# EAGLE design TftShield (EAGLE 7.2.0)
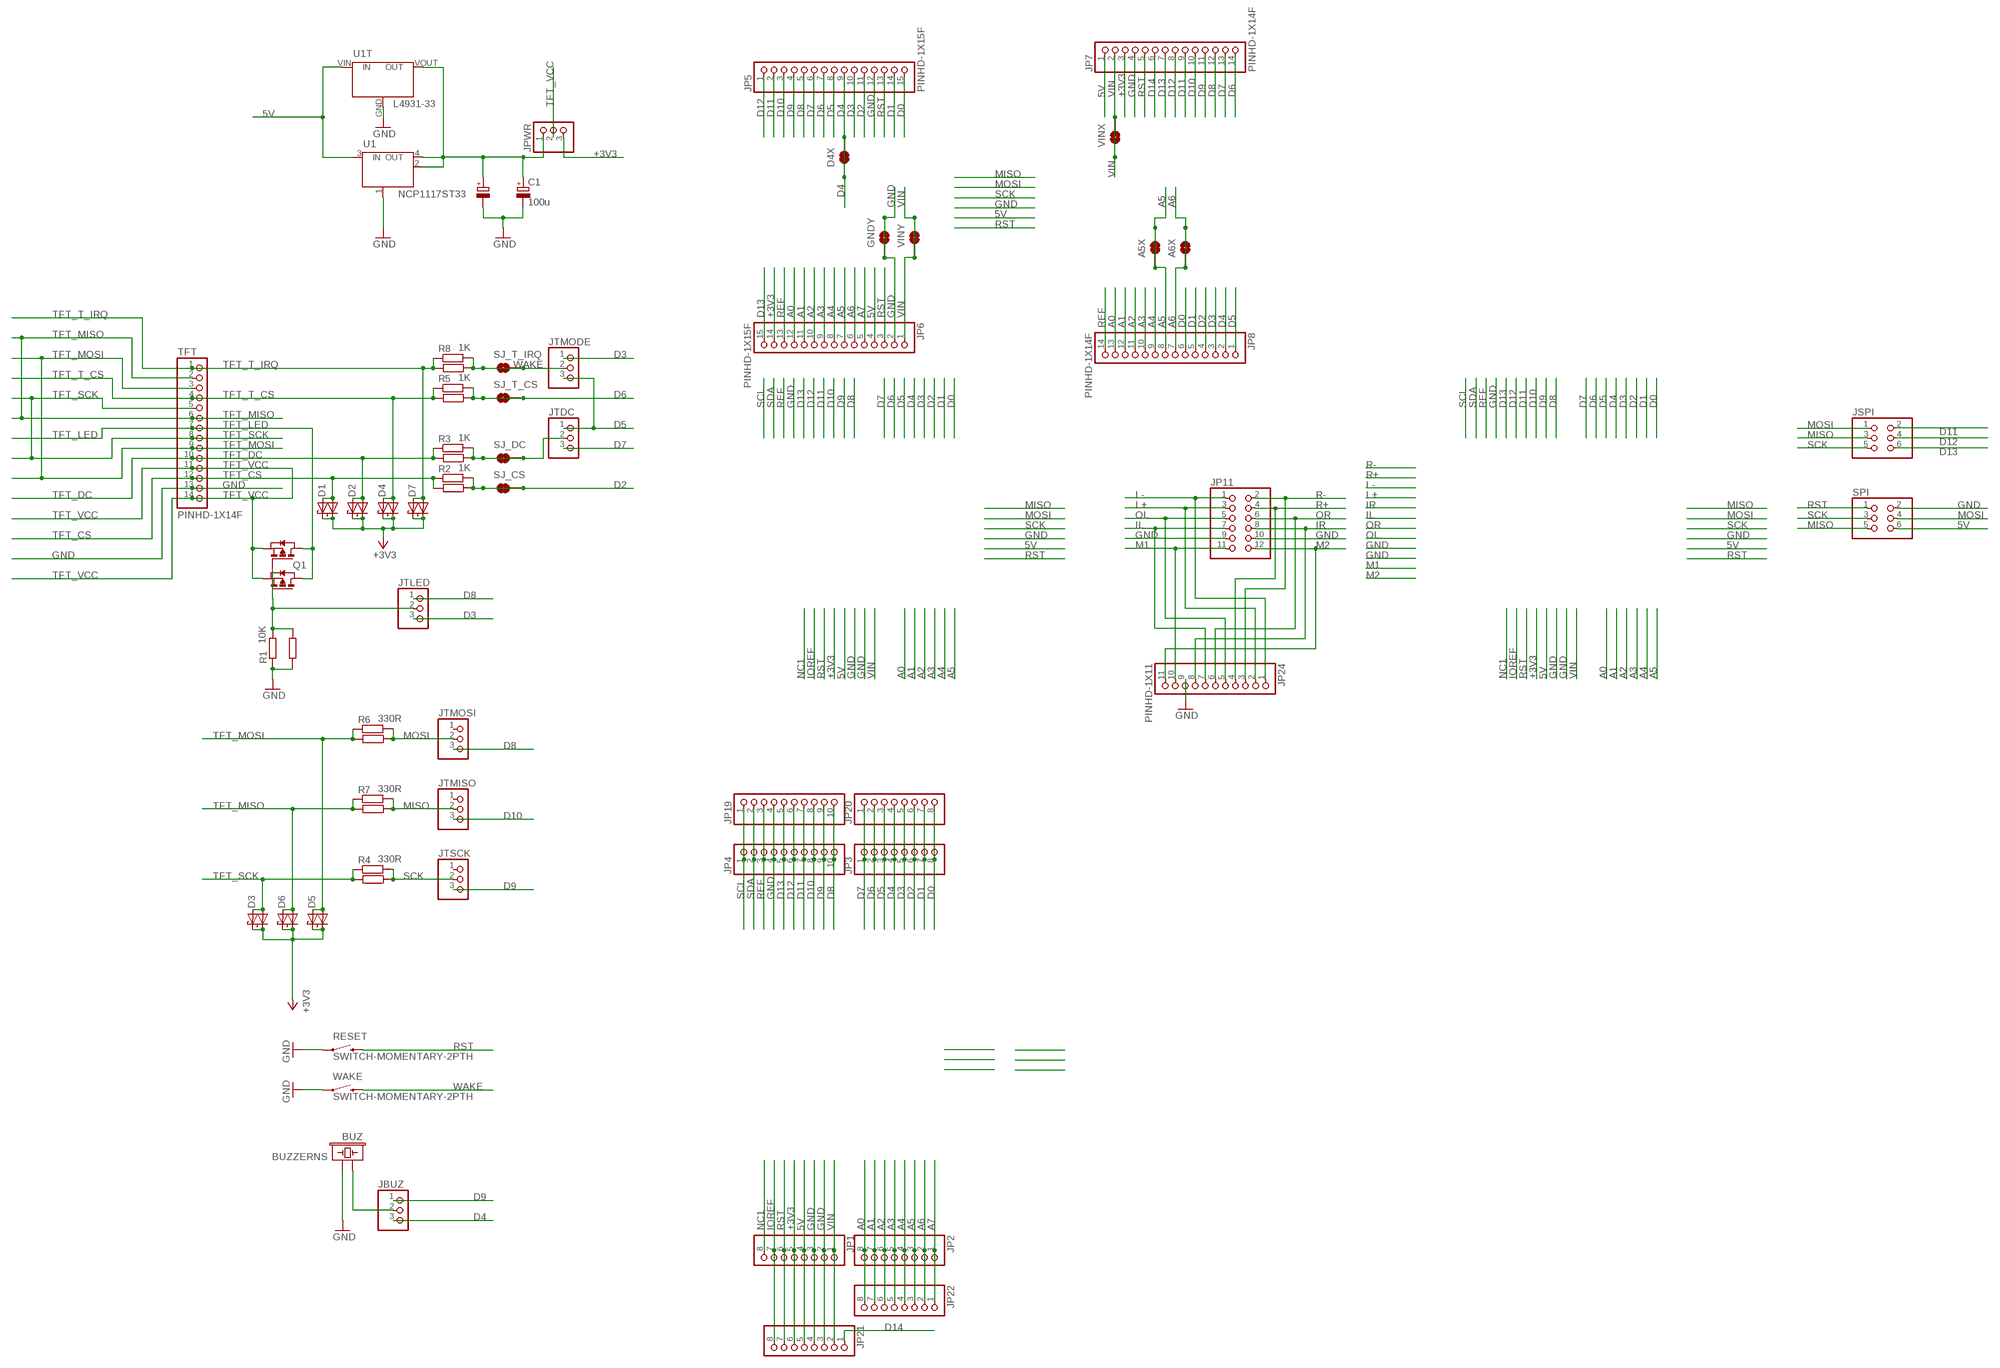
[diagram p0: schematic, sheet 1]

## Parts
A5X  JUMPER-PAD-2-NOYES_SILK  [PAD-JUMPER-2-NO_YES_SILK]
A6X  JUMPER-PAD-2-NOYES_SILK  [PAD-JUMPER-2-NO_YES_SILK]
BUZ  BUZZERNS  [BUZZER-12MM-NS]
C1  100u  CPOLPANASONIC_E  [PANASONIC_E]
C1T  CPOL-EUE3.5-8  [E3,5-8]
D1  RB521S  [SOD523]
D1T  1N4148DO35-7  [DO35-7]
D2  RB521S  [SOD523]
D2T  1N4148DO35-7  [DO35-7]
D3  RB521S  [SOD523]
D3T  1N4148DO35-7  [DO35-7]
D4  RB521S  [SOD523]
D4T  1N4148DO35-7  [DO35-7]
D4X  JUMPER-PAD-2-NOYES_SILK  [PAD-JUMPER-2-NO_YES_SILK]
D5  RB521S  [SOD523]
D5T  1N4148DO35-7  [DO35-7]
D6  RB521S  [SOD523]
D6T  1N4148DO35-7  [DO35-7]
D7  RB521S  [SOD523]
D7T  1N4148DO35-7  [DO35-7]
GNDY  JUMPER-PAD-2-NOYES_SILK  [PAD-JUMPER-2-NO_YES_SILK]
JBUZ  PINHD-1X3  [1X03M]
JP1  PINHD-1X8  [1X08M]
JP2  PINHD-1X8  [1X08M]
JP3  PINHD-1X8  [1X08M]
JP4  PINHD-1X10  [1X10M]
JP5  PINHD-1X15F  [1X15F]
JP6  PINHD-1X15F  [1X15F]
JP7  PINHD-1X14F  [1X14F]
JP8  PINHD-1X14F  [1X14F]
JP11  PINHD-2X6F  [2X06F]
JP19  PINHD-1X10  [1X10M]
JP20  PINHD-1X8  [1X08M]
JP21  PINHD-1X8  [1X08M]
JP22  PINHD-1X8  [1X08M]
JP24  PINHD-1X11  [1X11M]
JPWR  PINHD-1X3  [1X03M]
JSPI  PINHD-2X3  [2X03M]
JTDC  PINHD-1X3  [1X03M]
JTLED  PINHD-1X3  [1X03M]
JTMISO  PINHD-1X3  [1X03M]
JTMODE  PINHD-1X3  [1X03M]
JTMOSI  PINHD-1X3  [1X03M]
JTSCK  PINHD-1X3  [1X03M]
Q1  PMOSSOT23  [SOT23]
Q1T  BS170  [TO92-MOSFET]
R1  10K  R0603-ROUND  [R0603-ROUND]
R1T  R0204-5  [0204-5]
R2  1K  R0603-ROUND  [R0603-ROUND]
R2T  R0204-5  [0204-5]
R3  1K  R0603-ROUND  [R0603-ROUND]
R3T  R0204-5  [0204-5]
R4  330R  R0603-ROUND  [R0603-ROUND]
R4T  R0204-5  [0204-5]
R5  1K  R0603-ROUND  [R0603-ROUND]
R5T  R0204-5  [0204-5]
R6  330R  R0603-ROUND  [R0603-ROUND]
R6T  R0204-5  [0204-5]
R7  330R  R0603-ROUND  [R0603-ROUND]
R7T  R0204-5  [0204-5]
R8  1K  R0603-ROUND  [R0603-ROUND]
R8T  R0204-5  [0204-5]
RESET  SWITCH-MOMENTARY-2PTH  [TACTILE-PTH]
SJ_CS  JUMPER-PAD-2-NOYES_SILK  [PAD-JUMPER-2-NO_YES_SILK]
SJ_DC  JUMPER-PAD-2-NOYES_SILK  [PAD-JUMPER-2-NO_YES_SILK]
SJ_T_CS  JUMPER-PAD-2-NOYES_SILK  [PAD-JUMPER-2-NO_YES_SILK]
SJ_T_IRQ  JUMPER-PAD-2-NOYES_SILK  [PAD-JUMPER-2-NO_YES_SILK]
SPI  PINHD-2X3F  [2X03F]
TFT  PINHD-1X14F  [1X14F]
U1  NCP1117ST33  [SOT223]
U1T  L4931-33  [TO92]
VINX  JUMPER-PAD-2-NOYES_SILK  [PAD-JUMPER-2-NO_YES_SILK]
VINY  JUMPER-PAD-2-NOYES_SILK  [PAD-JUMPER-2-NO_YES_SILK]
WAKE  SWITCH-MOMENTARY-2PTH  [TACTILE-PTH]

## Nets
5V: JP1.4 JP6.4 JP7.1 JP21.5 SPI.6 U1.3(IN) U1T.VIN(IN)
+3V3: D1.C D1T.C D2.C D2T.C D3.C D3T.C D4.C D4T.C D5.C D5T.C D6.C D6T.C D7.C D7T.C JP1.5 JP6.14 JP7.3 JP21.6 JPWR.3
A0: JP2.8 JP6.12 JP8.13 JP22.8
A1: JP2.7 JP6.11 JP8.12 JP22.7
A2: JP2.6 JP6.10 JP8.11 JP22.6
A3: JP2.5 JP6.9 JP8.10 JP22.5
A4: JP2.4 JP6.8 JP8.9 JP22.4
A5: A5X.1 A5X.2 JP2.3 JP6.7 JP8.8 JP22.3
A6: A6X.1 A6X.2 JP2.2 JP6.6 JP8.7 JP22.2
A7: JP2.1 JP6.5 JP22.1
D0: JP3.8 JP5.15 JP8.6 JP20.8
D1: JP3.7 JP5.14 JP8.5 JP20.7
D2: JP3.6 JP5.11 JP8.4 JP20.6 R2.2 R2T.1 SJ_CS.1 SJ_CS.2
D3: JP3.5 JP5.10 JP8.3 JP20.5 JTLED.3 JTMODE.1
D4: D4X.1 D4X.2 JBUZ.3 JP3.4 JP5.9 JP8.2 JP20.4
D5: JP3.3 JP5.8 JP8.1 JP20.3 JTDC.1 JTMODE.3
D6: JP3.2 JP5.7 JP7.14 JP20.2 R5.2 R5T.1 SJ_T_CS.1 SJ_T_CS.2
D7: JP3.1 JP5.6 JP7.13 JP20.1 JTDC.3
D8: JP4.10 JP5.5 JP7.12 JP19.10 JTLED.1 JTMOSI.3
D9: JBUZ.1 JP4.9 JP5.4 JP7.11 JP19.9 JTSCK.3
D10: JP4.8 JP5.3 JP7.10 JP19.8 JTMISO.3
D11: JP4.7 JP5.2 JP7.9 JP19.7 JSPI.2
D12: JP4.6 JP5.1 JP7.8 JP19.6 JSPI.4
D13: JP4.5 JP6.15 JP7.7 JP19.5 JSPI.6
D14: JP7.6 JP21.1
GND: BUZ.- C1.- C1T.- GNDY.1 GNDY.2 JP1.2 JP1.3 JP4.4 JP5.12 JP6.2 JP7.4 JP11.9 JP11.10 JP19.4 JP21.3 JP21.4 JP24.9 R1.1 R1T.1 RESET.1 RESET.2 SPI.2 TFT.13 U1.1(GND/ADJ) U1T.GND(GND/ADJ) WAKE.1 WAKE.2
IL: JP11.7 JP24.7
IOREF: JP1.7 JP21.8
IR: JP11.8 JP24.8
L+: JP11.3 JP24.2
L-: JP11.1 JP24.1
M1: JP11.11 JP24.10
M2: JP11.12 JP24.11
MISO: JSPI.3 JTMISO.2 R7.2 R7T.1 SPI.5
MOSI: JSPI.1 JTMOSI.2 R6.2 R6T.1 SPI.4
N$2: BUZ.+ JBUZ.2
N$4: JTLED.2 Q1.1(G) Q1T.G R1.2 R1T.2
N$5: JTDC.2 R3.2 R3T.1 SJ_DC.1 SJ_DC.2
N$10: C1.+ C1T.+ JPWR.1 U1.2(OUT) U1.4(OUT) U1T.VOUT(OUT)
NC1: JP1.8
OL: JP11.5 JP24.5
OR: JP11.6 JP24.6
R+: JP11.4 JP24.4
R-: JP11.2 JP24.3
REF: JP4.3 JP6.13 JP8.14 JP19.3
RST: JP1.6 JP5.13 JP6.3 JP7.5 JP21.7 RESET.3 RESET.4 SPI.1
SCK: JSPI.5 JTSCK.2 R4.2 R4T.1 SPI.3
SCL: JP4.1 JP19.1
SDA: JP4.2 JP19.2
TFT_CS: D1.A D1T.A R2.1 R2T.2 TFT.12
TFT_DC: D2.A D2T.A R3.1 R3T.2 TFT.10
TFT_LED: Q1.3(D) Q1T.D TFT.7
TFT_MISO: D6.A D6T.A R7.1 R7T.2 TFT.2 TFT.6
TFT_MOSI: D5.A D5T.A R6.1 R6T.2 TFT.3 TFT.9
TFT_SCK: D3.A D3T.A R4.1 R4T.2 TFT.5 TFT.8
TFT_T_CS: D4.A D4T.A R5.1 R5T.2 TFT.4
TFT_T_IRQ: D7.A D7T.A R8.1 R8T.2 TFT.1
TFT_VCC: JPWR.2 Q1.2(S) Q1T.S TFT.11 TFT.14
VIN: JP1.1 JP6.1 JP7.2 JP21.2 VINX.1 VINX.2 VINY.1 VINY.2
WAKE: JTMODE.2 R8.2 R8T.1 SJ_T_IRQ.1 SJ_T_IRQ.2 WAKE.3 WAKE.4
Unconnected: JTMISO.1 JTMOSI.1 JTSCK.1

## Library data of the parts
A5X A6X D4X GNDY SJ_CS SJ_DC SJ_T_CS SJ_T_IRQ VINX VINY = Max-Connectors:JUMPER-PAD-2-NO
BUZ = Max-Buzzers:BUZZER: Buzzer 12mm
C1 = Max-RCL:CPOL
C1T = rcl:CPOL-EU: POLARIZED CAPACITOR, European symbol
D1-D7 = Max-Diodes:RB521S
D1T D2T D3T D4T D5T D6T D7T = Max-Diodes:1N4148: DIODE
JBUZ JPWR JTDC JTLED JTMISO JTMODE JTMOSI JTSCK = Max-PinHead:PINHD-1X3: PIN HEADER
JP1-JP3 JP20-JP22 = Max-PinHead:PINHD-1X8: PIN HEADER
JP4 JP19 = Max-PinHead:PINHD-1X10: PIN HEADER
JP5 JP6 = Max-PinHead:PINHD-1X15
JP7 JP8 TFT = Max-PinHead:PINHD-1X14
JP11 = Max-PinHead:PINHD-2X6
JP24 = Max-PinHead:PINHD-1X11
JSPI SPI = Max-PinHead:PINHD-2X3: PIN HEADER
Q1 = Max-Mosfets:PMOSSOT23: MOS FET
Q1T = Max-Mosfets:BS170
R1 R1T R2 R2T R3 R3T R4 R4T R5 R5T R6 R6T R7 R7T R8 R8T = Max-RCL:R
RESET WAKE = Max-Switches:SWITCH-MOMENTARY-2: Various NO switches- pushbuttons, reed, etc; PROD_ID: SWCH-08441
U1 = Max-LinearRegulators:NCP1117: Adjustable Output Low Dropout Voltage Regulator 800 mA Source: http://www.onsemi.com/pub/Collateral/MC33269-D.PDF
U1T = Max-LinearRegulators:L4931-33

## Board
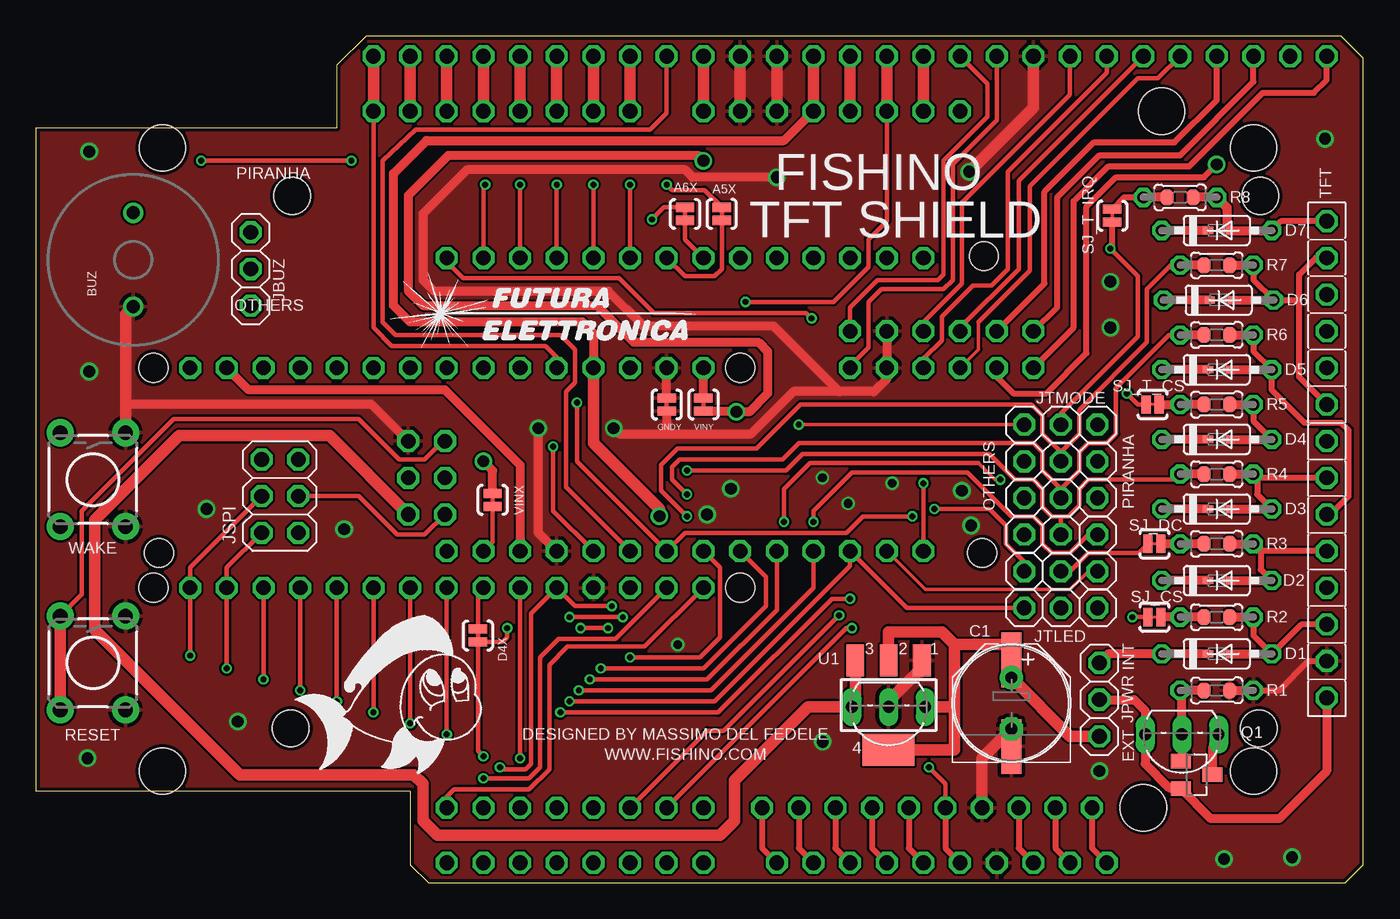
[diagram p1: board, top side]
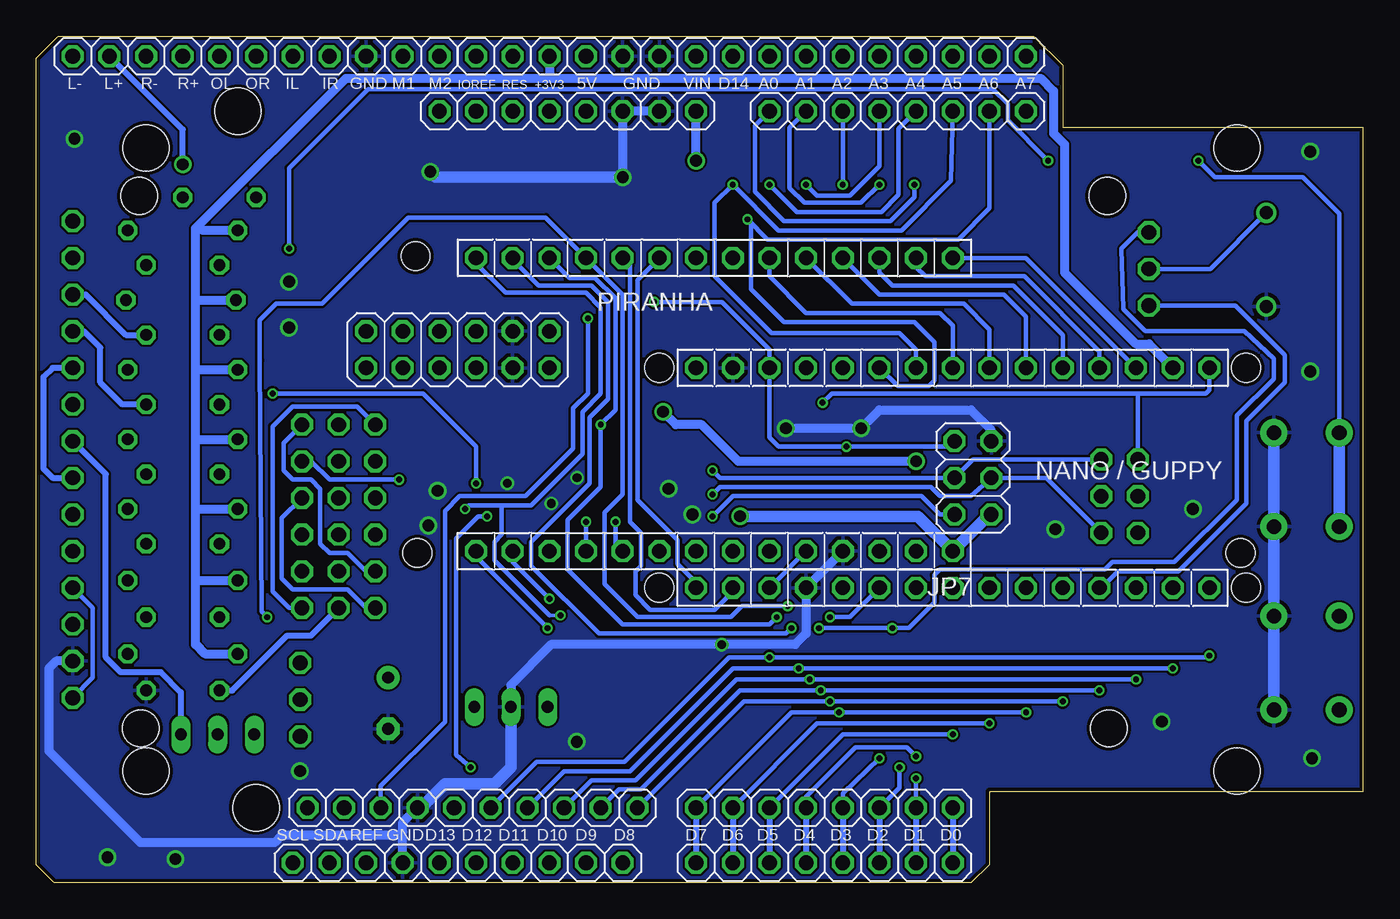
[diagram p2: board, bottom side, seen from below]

Size 91.95 x 58.67 mm. Coordinates in mm from the lower left corner, seen from the top.
Outline: 25.91,6.35 25.91,1.27 27.18,0 90.68,0 91.95,1.27 91.95,57.15 90.42,58.67 22.86,58.67 20.83,56.64 20.83,52.32 0,52.32 0,6.35 25.91,6.35
Copper layers (1*16): Top 0.035mm / dielectric 1.5mm / Bottom 0.035mm
Design rules "Elecrow_2-layer_eagle_rule": minimum track width 6mil, minimum drill 12mil, track to track 6mil, track to pad 6mil, pad to pad 6mil, via to via 6mil, smd to smd 0mil, copper to edge 10mil, drill to drill 10mil, minimum pad ring 10mil, minimum via ring 6mil, stop-mask expansion 2mil, vias tented up to drill 100mil, thermal gap 10mil
Holes 3.2 mm at 84.33,7.75 8.76,7.75 8.76,50.93 84.33,50.93 76.71,5.21 77.98,53.47
Holes 2 mm at 8.13,20.45 8.51,22.86 8.13,35.69 48.77,20.45 48.77,35.69 65.53,22.86 65.66,43.43
Holes 2.54 mm at 17.73,47.6 17.63,10.72 84.71,10.72 84.81,47.6

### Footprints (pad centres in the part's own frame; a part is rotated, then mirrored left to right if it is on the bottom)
PAD-JUMPER-2-NO_YES_SILK = smd 0.635 x 1.27: 1 -0.45,0; 2 0.45,0
BUZZER-12MM-NS = drill 0.9: + 3.25,0; - -3.25,0
PANASONIC_E = smd 3.8 x 1.4: + 3,0; - -3,0
E3,5-8 = drill 0.813 pad 1.6: + -1.778,0 | drill 0.813 pad 1.6 octagon: - 1.778,0
SOD523 = smd 0.7 x 0.5: A 0.7,0; C -0.6,0
DO35-7 = drill 0.813 octagon: A 3.81,0; C -3.81,0
1X03M = drill 1.016 octagon: 1 -2.54,0; 2 0,0; 3 2.54,0
1X08M = drill 1.016 octagon: 1 -8.89,0; 2 -6.35,0; 3 -3.81,0; 4 -1.27,0; 5 1.27,0; 6 3.81,0; 7 6.35,0; 8 8.89,0
1X10M = drill 1.016 octagon: 1 -11.43,0; 2 -8.89,0; 3 -6.35,0; 4 -3.81,0; 5 -1.27,0; 6 1.27,0; 7 3.81,0; 8 6.35,0; 9 8.89,0; 10 11.43,0
1X15F = drill 1.016 octagon: 1 -17.78,0; 2 -15.24,0; 3 -12.7,0; 4 -10.16,0; 5 -7.62,0; 6 -5.08,0; 7 -2.54,0; 8 0,0; 9 2.54,0; 10 5.08,0; 11 7.62,0; 12 10.16,0; 13 12.7,0; 14 15.24,0; 15 17.78,0
1X14F = drill 1.016 octagon: 1 -16.51,0; 2 -13.97,0; 3 -11.43,0; 4 -8.89,0; 5 -6.35,0; 6 -3.81,0; 7 -1.27,0; 8 1.27,0; 9 3.81,0; 10 6.35,0; 11 8.89,0; 12 11.43,0; 13 13.97,0; 14 16.51,0
2X06F = drill 1.016 octagon: 1 -6.35,-1.27; 2 -6.35,1.27; 3 -3.81,-1.27; 4 -3.81,1.27; 5 -1.27,-1.27; 6 -1.27,1.27; 7 1.27,-1.27; 8 1.27,1.27; 9 3.81,-1.27; 10 3.81,1.27; 11 6.35,-1.27; 12 6.35,1.27
1X11M = drill 1.016 octagon: 1 -12.7,0; 2 -10.16,0; 3 -7.62,0; 4 -5.08,0; 5 -2.54,0; 6 0,0; 7 2.54,0; 8 5.08,0; 9 7.62,0; 10 10.16,0; 11 12.7,0
2X03M = drill 1.016 octagon: 1 -2.54,-1.27; 2 -2.54,1.27; 3 0,-1.27; 4 0,1.27; 5 2.54,-1.27; 6 2.54,1.27
SOT23 = smd 1 x 1.4: 1 -0.95,-1.1; 2 0.95,-1.1; 3 0,1.1
TO92-MOSFET = drill 0.813 long: D -2.54,0; G 0,0; S 2.54,0
R0603-ROUND = smd 0.898 x 1.1: 1 -0.889,0; 2 0.889,0
0204-5 = drill 0.813 octagon: 1 -2.54,0; 2 2.54,0
TACTILE-PTH = drill 1.016 pad 1.88: 1 -3.251,2.261; 2 3.251,2.261; 3 -3.251,-2.261; 4 3.251,-2.261
2X03F = drill 1.016 octagon: 1 -2.54,-1.27; 2 -2.54,1.27; 3 0,-1.27; 4 0,1.27; 5 2.54,-1.27; 6 2.54,1.27
SOT223 = smd 1.219 x 2.235: 1 -2.311,-3.099; 2 0,-3.099; 3 2.311,-3.099 | smd 3.6 x 2.2: 4 0,3.099
TO92 = drill 0.813 long: GND 0,0; VIN 2.54,0; VOUT -2.54,0

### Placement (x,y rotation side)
A5X  47.5,46.35 90 top
A6X  44.96,46.35 90 top
BUZ  6.73,43.18 90 top
C1  67.56,12.45 90 top
C1T  67.56,12.45 270 top
D1  81.79,15.88 0 top
D1T  81.79,15.88 0 top
D2  81.79,20.95 0 top
D2T  81.79,20.95 0 top
D3  81.79,25.91 0 top
D3T  81.79,25.91 0 top
D4  81.79,30.73 0 top
D4T  81.79,30.73 0 top
D4X  30.61,17.14 90 top
D5  81.79,35.56 0 top
D5T  81.79,35.56 0 top
D6  81.92,40.39 0 top
D6T  81.92,40.39 0 top
D7  81.79,45.21 0 top
D7T  81.79,45.21 0 top
GNDY  43.69,33.15 270 top
JBUZ  14.86,42.55 90 top
JP1  55.12,53.47 180 bottom
JP2  32.26,53.47 180 bottom
JP3  37.34,5.21 0 bottom
JP4  61.72,5.21 0 bottom
JP5  28.45,20.45 180 bottom
JP6  28.45,35.69 0 bottom
JP7  44.96,22.99 180 bottom
JP8  44.96,43.31 0 bottom
JP11  62.74,36.96 0 bottom
JP19  62.74,1.4 0 bottom
JP20  37.34,1.4 0 bottom
JP21  52.58,57.28 180 bottom
JP22  32.26,57.28 180 bottom
JP24  76.71,57.28 0 bottom
JPWR  73.66,12.7 90 top
JSPI  16.89,26.8 90 top
JTDC  70.99,21.59 0 top
JTLED  70.99,19.05 0 top
JTMISO  70.99,29.21 0 top
JTMODE  70.99,31.75 0 top
JTMOSI  70.99,26.67 0 top
JTSCK  70.99,24.13 0 top
Q1  80.39,7.49 270 top
Q1T  79.38,10.29 180 top
R1  81.79,13.34 180 top
R1T  81.79,13.34 180 top
R2  81.79,18.41 180 top
R2T  81.79,18.41 0 top
R3  81.79,23.5 180 top
R3T  81.79,23.5 0 top
R4  81.79,28.32 180 top
R4T  81.79,28.32 0 top
R5  81.79,33.15 180 top
R5T  81.79,33.15 0 top
R6  81.79,37.97 180 top
R6T  81.79,37.97 0 top
R7  81.79,42.8 180 top
R7T  81.79,42.8 0 top
R8  79.25,47.5 180 top
R8T  79.25,47.5 0 top
RESET  3.94,15.24 270 top
SJ_CS  77.47,18.41 180 top
SJ_DC  77.47,23.5 180 top
SJ_T_CS  77.34,33.15 180 top
SJ_T_IRQ  74.55,46.23 270 top
SPI  27.05,28.07 270 bottom
TFT  89.41,29.34 270 top
U1  59.05,12.32 180 top
U1T  59.05,12.19 180 top
U$3  [FISHINO]  19.68,7.87 0 top
U$5  [FUTURA]  24.38,37.08 0 top
VINX  31.62,26.54 270 top
VINY  46.23,33.15 270 top
WAKE  3.94,27.94 270 top

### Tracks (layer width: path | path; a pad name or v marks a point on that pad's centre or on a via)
5V  (via drill 0.81)
  Top 0.61: JP6.4 38.61,38.1 37.85,38.86 25.91,38.86 24.77,40.01 24.77,49.15 27.05,51.44 51.82,51.44 JP1.4
  Top 0.813: U1.3 56.74,12.42 U1T.VIN 53.47,12.19 48.39,7.11 48.39,4.32 47.37,3.3 27.81,3.3 26.8,4.32 26.8,6.86 26.16,7.49 14.1,7.49 4.06,17.53 4.06,25.15 9.91,30.99 20.32,30.99 SPI.6 | JP1.4 JP21.5 | v43.18,25.4 43.18,25.91 38.61,30.48 JP6.4
  Bottom 0.813: v43.18,25.4 30.86,25.4 JP7.1 25.91,25.53 SPI.6
+3V3
  Top 0.61: JP7.3 33.53,28.96 28.32,34.16 14.73,34.16 JP6.14 | D7.C D7T.C | D6.C D6T.C | D5.C D5T.C | D4.C D4T.C | D3.C D3T.C | D1.C D1T.C 74.3,15.88 JPWR.3 | D2.C D2T.C
  Top 0.813: JP1.5 JP21.6
  Bottom 0.61: 56.39,55.75 22.35,55.75 21.46,54.86 21.46,51.94 20.7,51.18 20.7,42.29 15.75,37.34 14.86,37.34 JP6.14 | D1T.C 80.26,15.88 80.9,16.51 80.9,20.95 | 80.9,20.95 D2T.C | 80.9,20.95 80.9,25.91 | 80.9,25.91 D3T.C | 80.9,25.91 80.9,30.73 | 80.9,30.73 D4T.C | 80.9,30.73 80.9,35.56 | 80.9,35.56 D5T.C | 80.9,35.56 80.9,40.39 | 80.9,40.39 D6T.C | 80.9,40.39 80.9,45.34 80.71,45.53 | JP21.6 56.39,55.75 | D7T.C 80.39,45.21 80.71,45.53 | 80.71,45.53 70.48,55.75 56.39,55.75
A0  (via drill 0.41)
  Top 0.305: JP8.13 30.99,48.26 v31.11,48.39
  Top 0.813: JP2.8 JP22.8
  Bottom 0.305: JP2.8 42.16,52.45 42.16,47.88 40.13,45.85 32.77,45.85 31.11,47.5 v31.11,48.39 | JP8.13 30.99,42.67 30.35,42.04 23.5,42.04 18.29,36.83 JP6.12
A1  (via drill 0.41)
  Top 0.305: JP8.12 v33.53,48.39
  Top 0.813: JP2.7 JP22.7
  Bottom 0.305: JP2.7 39.75,52.32 39.75,48.13 38.73,47.12 34.8,47.12 v33.53,48.39 | JP8.12 33.53,42.29 32.64,41.4 24.26,41.4 20.83,37.97 JP6.11
A2  (via drill 0.41)
  Top 0.305: v36.07,48.39 JP8.11
  Top 0.813: JP2.6 JP22.6
  Bottom 0.305: JP2.6 v36.07,48.39 | JP8.11 33.53,40.77 24.89,40.77 23.37,39.24 JP6.10
A3  (via drill 0.41)
  Top 0.305: JP8.10 v38.61,48.39
  Top 0.813: JP2.5 JP22.5
  Bottom 0.305: JP2.5 33.53,49.66 35.56,47.62 37.85,47.62 v38.61,48.39 | JP6.9 25.91,38.35 27.69,40.13 35.43,40.13 JP8.10
A4  (via drill 0.41)
  Top 0.305: JP8.9 v41.15,48.39
  Top 0.813: JP2.4 JP22.4
  Bottom 0.305: JP2.4 32.19,52.26 32.19,47.69 33.4,46.48 39.24,46.48 v41.15,48.39 | JP6.8 28.45,38.61 29.34,39.5 38.61,39.5 41.15,42.04 JP8.9
A5  (via drill 0.41)
  Top 0.305: v43.69,48.39 44.07,48.01 46.3,48.01 A5X.2 A5X.1 47.5,42.55 46.99,42.04 44.96,42.04 JP8.8
  Top 0.813: JP2.3 JP22.3
  Bottom 0.305: JP2.3 28.57,48.64 32,45.21 40.51,45.21 v43.69,48.39 44.96,47.12 44.96,42.04 41.02,38.1 32.13,38.1 30.99,36.96 JP6.7
A6  (via drill 0.41)
  Top 0.305: v42.67,45.97 43.5,46.8 A6X.2 A6X.1 44.96,44.58 JP8.7
  Top 0.813: JP2.2 JP22.2
  Bottom 0.305: JP2.2 25.91,46.74 28.07,44.58 41.27,44.58 v42.67,45.97 42.42,45.72 42.42,41.15 40.13,38.86 31.11,38.86 29.72,37.47 29.72,34.8 30.1,34.42 32.26,34.42 JP6.6
A7
  Top 0.305: JP6.5 36.07,36.45 35.31,37.21 24.64,37.21 23.37,38.48 JP2.1
  Top 0.813: JP2.1 JP22.1
D0
  Top 0.305: JP5.15 42.16,16.38 36.83,16.38 35.56,15.11 35.56,7.87 34.16,6.48 28.96,6.48 28.45,5.97 JP3.8
  Bottom 0.305: JP5.15 46.23,20.83 47.5,22.1 47.5,23.75 50.29,26.54 50.29,41.78 JP8.6
  Bottom 0.406: JP3.8 JP20.8
D1  (via drill 0.41)
  Top 0.305: v30.99,7.24 34.16,7.24 34.92,8 34.92,15.62 36.2,16.89 40.13,16.89 JP5.14
  Bottom 0.305: JP3.7 v30.99,7.24 | JP5.14 43.69,20.19 44.96,18.92 49.4,18.92 50.42,19.94 50.42,21.59 50.04,21.97 50.04,24.26 50.8,25.02 50.8,42.8 JP8.5
  Bottom 0.406: JP3.7 JP20.7
D2  (via drill 0.41)
  Top 0.203: SJ_CS.2 SJ_CS.1
  Top 0.254: v32.13,8 32.26,7.87
  Top 0.305: 32.26,7.87 33.91,7.87 34.29,8.26 34.29,18.67 JP5.11 37.34,19.18 v39.88,19.18 | SJ_CS.2 v75.95,18.41
  Top 0.61: SJ_CS.1 R2T.1 R2.2
  Bottom 0.305: JP3.6 32.13,6.6 v32.13,8 | v39.88,19.18 43.05,19.18 43.81,18.41 50.29,18.41 52.58,20.7 52.58,25.65 51.31,26.92 51.31,40.77 JP8.4 56.64,46.1 66.17,46.1 72.14,40.13 75.31,40.13 76.45,38.99 76.45,36.2 76.33,18.8 v75.95,18.41
  Bottom 0.406: JP3.6 JP20.6
D3  (via drill 0.41)
  Top 0.254: JTMODE.1 v52.83,31.75
  Top 0.305: v33.53,8.64 JP5.10 | v40.64,18.41 v36.96,18.41
  Bottom 0.305: v33.53,8.64 36.07,6.22 JP3.5 | v40.64,18.41 41.15,17.91 51.31,17.91 55.12,21.72 55.12,25.15 52.83,27.43 v52.83,31.75 51.82,32.77 51.82,40.51 53.21,41.91 54.99,41.91 JP8.3 | v36.96,18.41 35.56,18.41 JP5.10 | JTLED.3 74.42,19.05 75.56,20.19 75.56,31.62 74.17,33.02 69.72,33.02 JTMODE.1
  Bottom 0.406: JP3.5 JP20.5
D4  (via drill 0.41)
  Top 0.305: v39.62,17.65 v37.72,17.65 | D4X.1 30.61,9.14 v30.99,8.76 | D4X.1 32.32,16.7 32.64,17.02 v32.64,17.65 | D4X.1 D4X.2 30.61,20.07 JP5.9
  Bottom 0.305: JP3.4 38.61,5.97 35.18,9.4 31.62,9.4 v30.99,8.76 | JP8.2 58.93,43.18 57.15,41.4 53.47,41.4 52.32,40.26 52.32,33.53 53.59,32.26 53.59,27.69 57.66,23.62 57.66,21.97 52.96,17.27 40.01,17.27 v39.62,17.65 | JBUZ.3 15.62,45.09 16.76,43.94 16.64,39.75 15.11,38.23 8.26,38.23 6.22,36.32 6.22,34.92 8.76,32.38 8.76,26.54 13.08,22.23 17.4,22.23 17.91,21.72 29.34,21.72 29.72,21.34 29.72,19.43 31.5,17.65 v32.64,17.65 v37.72,17.65
  Bottom 0.406: JP3.4 JP20.4
D5  (via drill 0.41)
  Top 0.305: JP5.8 v28.45,10.29 | v55.63,18.54 47.62,10.54 46.48,10.54 JP3.3 | JTDC.1 68.45,22.23 67.18,23.5 67.18,24.77 66.04,25.91 v62.23,25.91
  Bottom 0.254: 56.39,18.54 v55.63,18.54
  Bottom 0.305: v28.45,10.29 36.07,10.29 JP3.3 | JP8.1 61.47,42.93 59.44,40.89 53.85,40.89 52.83,39.88 52.83,33.91 54.1,32.64 54.1,29.72 57.66,26.16 59.69,26.16 | 56.39,18.54 60.2,22.35 60.2,23.62 59.69,24.13 59.69,26.16 | JTDC.1 69.09,21.59 70.36,22.86 71.63,22.86 72.26,23.5 72.26,27.3 72.9,27.94 74.17,27.94 74.8,28.57 74.8,30.48 JTMODE.3 | v62.23,25.91 61.98,26.16 59.69,26.16
  Bottom 0.406: JP3.3 JP20.3
D6  (via drill 0.41)
  Top 0.203: SJ_T_CS.1 SJ_T_CS.2
  Top 0.305: JP5.7 v25.91,11.05 | SJ_T_CS.2 76.33,33.15 v75.56,33.91 | JP3.2 56.13,17.65 v56.52,17.65 | v61.47,27.69 JP7.14
  Top 0.61: R5.2 R5T.1 SJ_T_CS.1
  Bottom 0.305: v25.91,11.05 37.85,11.05 JP3.2 | v75.56,33.91 65.15,33.91 61.47,30.23 v61.47,27.69 | v56.52,17.65 61.47,22.61 JP7.14
  Bottom 0.406: JP3.2 JP20.2
D7  (via drill 0.41)
  Top 0.254: JTDC.3 72.9,21.59 71.63,20.32 61.59,20.32 JP7.13
  Top 0.305: JP5.6 v23.37,11.81 | v56.39,19.68 55.12,19.68 47.24,11.81 v36.32,11.81
  Bottom 0.305: v23.37,11.81 v36.32,11.81 39.62,11.81 JP3.1 | JP7.13 58.93,22.23 v56.39,19.68
  Bottom 0.406: JP3.1 JP20.1
D8  (via drill 0.41)
  Top 0.305: JP5.5 v20.83,12.57 | JTLED.1 60.33,19.05 JP7.12 56.39,21.97 46.99,12.57 v36.96,12.57
  Top 0.406: JP4.10 50.29,2.41 JP19.10
  Bottom 0.305: v20.83,12.57 v36.96,12.57 42.93,12.57 JP4.10 | JTLED.1 69.09,19.05 70.36,20.32 74.17,20.32 74.93,21.08 74.93,25.27 JTMOSI.3
D9  (via drill 0.41)
  Top 0.305: JP5.4 v18.29,13.34 | JTSCK.3 72.9,24.13 71.63,22.86 70.36,22.86 69.72,23.5 69.72,24.77 69.09,25.4 67.56,25.4 64.52,28.45 56.52,28.45 53.85,25.78 v53.85,25.02 | JP7.11 53.85,20.45 46.74,13.34 v37.59,13.34
  Top 0.406: JP4.9 52.83,2.41 JP19.9
  Bottom 0.254: 52.7,5.21 JP4.9
  Bottom 0.305: v18.29,13.34 v37.59,13.34 43.18,13.34 50.04,6.48 51.56,6.48 JP4.9 | JP7.11 v53.85,25.02 | JP5.4 18.16,20.45 17.02,21.59 12.83,21.59 8.13,26.29 8.13,32 5.46,34.67 5.46,36.58 8.89,40.01 JBUZ.1
D10  (via drill 0.41)
  Top 0.254: v66.8,27.94 66.42,27.94 65.28,29.08
  Top 0.305: JP5.3 v15.75,14.1 | 65.28,29.08 53.59,29.08 51.82,27.3 v51.82,25.02 | JP7.10 51.31,18.92 46.48,14.1 v38.35,14.1
  Top 0.406: JP4.8 55.37,2.41 JP19.8
  Bottom 0.305: v15.75,14.1 v38.35,14.1 43.43,14.1 50.42,7.11 53.47,7.11 JP4.8 | JTMISO.3 72.9,29.21 71.63,27.94 v66.8,27.94 | JP7.10 51.82,23.5 v51.82,25.02
D11  (via drill 0.41)
  Top 0.305: v13.21,14.86 JP5.2 13.21,21.84 JSPI.2 | JP7.9 50.55,21.21 50.55,19.18 46.23,14.86 v39.12,14.86
  Top 0.406: JP4.7 57.91,2.41 JP19.7
  Bottom 0.305: v13.21,14.86 v39.12,14.86 43.69,14.86 50.8,7.75 55.37,7.75 JP4.7
D12  (via drill 0.41)
  Top 0.305: v10.67,15.75 JP5.1 10.67,21.84 JSPI.4 | JP7.8 47.37,21.84 47.37,17.02 45.97,15.62 v41.15,15.62
  Top 0.406: JP4.6 60.45,2.41 JP19.6
  Bottom 0.254: v10.67,15.75 10.79,15.62
  Bottom 0.305: 10.79,15.62 v41.15,15.62 43.94,15.62 51.18,8.38 57.28,8.38 JP4.6
D13  (via drill 0.41)
  Top 0.305: v37.47,33.27 37.47,29.21 JP7.7 44.96,24.26 56.13,24.26 57.28,25.4 v60.71,25.4 | v61.85,8 62.99,6.86 JP4.5
  Top 0.406: JP4.5 62.99,2.41 JP19.5
  Bottom 0.254: 15.62,33.78 15.75,33.91
  Bottom 0.305: JP6.15 10.67,34.16 10.92,33.91 15.75,33.91 36.83,33.91 v37.47,33.27 | v60.71,25.4 61.34,25.4 62.87,23.88 62.87,8.89 v61.85,8 | JSPI.6 15.62,33.78
D14
  Top 0.305: JP7.6 36.7,27.43 36.7,34.04 37.34,34.67 37.34,36.96 36.32,37.97 24.89,37.97 24,38.86 24,50.04 26.29,52.2 42.55,52.2 43.69,53.34 JP21.1
GND  (via drill 0.61, 0.81)
  Top 0.305: GNDY.1 GNDY.2
  Top 0.406: R1T.1 86.11,13.34 88.14,15.37 TFT.13
  Top 0.61: JP11.10 JP11.9 58.93,34.92 58.04,34.04 55.63,34.04 | JP7.4 34.8,24.26 v34.8,31.5 | R1.1 R1T.1 | 55.63,34.04 52.45,34.04 49.53,31.11 43.56,31.11 | SPI.2 23.24,33.15 6.2,33.15 | v51.31,48.9 45.47,48.9 44.96,49.4 29.84,49.4 26.8,46.35 26.8,41.78 27.56,41.02 39.62,41.02 42.04,38.61 51.05,38.61 55.63,34.04 | v40.01,31.5 40.39,31.11 43.56,31.11 | GNDY.2 43.69,31.24 43.56,31.11 | GNDY.1 JP6.2
  Top 0.813: C1.- C1T.- 65.53,8.64 JP4.4 | U1T.GND 59.05,12.57 61.34,14.86 61.34,15.39 U1.1 | JP24.9 69.09,53.72 v64.64,49.28 | WAKE.1 6.2,33.15 6.2,39.4 BUZ.- | JP1.3 JP21.4 | JP21.3 JP1.2
  Bottom 0.61: JP7.4 JP5.12 38.61,17.27 39.37,16.51 56.26,16.51 59.05,13.72 U1T.GND | SPI.2 25.78,31.37 27.18,32.77 33.53,32.77 v34.8,31.5 v40.01,31.5 | JP1.2 JP1.3 v51.31,48.9 | 65.28,5.21 JP4.4 66.55,4.19 66.55,3.56 | JP19.4 66.55,3.56 | 66.55,3.56 66.8,3.3 74.93,3.3 75.44,2.79 84.71,2.79 91.06,9.14 91.06,14.86 90.55,15.37 TFT.13
  Bottom 0.813: 65.28,5.21 63.63,6.86 60.2,6.86 59.05,8 U1T.GND | WAKE.1 WAKE.2 RESET.1 RESET.2 | v51.31,48.9 64.26,48.9 v64.64,49.28
  other vias: 59.31,27.69 56.26,26.29 87,1.78 82.3,1.65 89.28,51.56 3.68,35.43 3.68,50.67 21.34,24.51 11.81,25.91 13.97,11.18 3.56,8.64 54.48,9.78 73.66,7.75 54.48,28.07 44.45,16.51 48.13,27.3 46.48,25.53 64.14,27.18 64.77,24.77 74.42,41.66 74.42,38.48
  pour Bottom: 0,0 91.95,0 91.95,58.8 0,58.8
  pour Top: 0,0 91.95,0 91.95,58.67 0,58.67
IL
  Top 0.305: JP11.7 61.47,36.32 62.74,37.59 62.74,39.24 64.9,41.4 66.17,41.4 67.31,42.55 67.31,49.28 74.17,56.13 JP24.7
IOREF
  Top 0.813: JP1.7 JP21.8
IR
  Top 0.305: JP11.8 61.47,38.86 64.14,41.53 64.14,47.12 71.63,54.61 JP24.8
L+  (via drill 0.81)
  Top 0.406: JP11.3 66.55,35.05 67.69,33.91 69.98,33.91 72.77,36.7 72.77,46.86 74.8,48.9 80.9,48.9 v81.79,49.78
  Bottom 0.406: v81.79,49.78 81.79,52.2 JP24.2
L-
  Top 0.406: JP11.1 71.88,38.48 71.88,47.24 74.3,49.66 79.88,49.66 84.96,54.74 88.52,54.74 89.41,55.63 JP24.1
M1
  Top 0.305: JP11.11 56.39,35.81 57.66,37.08 57.66,40.26 58.55,41.15 62.87,41.15 63.5,41.78 63.5,49.78 66.55,52.83 JP24.10
M2
  Top 0.305: JP11.12 56.39,39.88 58.29,41.78 62.48,41.78 62.87,42.16 62.87,50.04 65.91,53.09 65.91,55.37 JP24.11
MISO  (via drill 0.41)
  Top 0.305: JTMISO.2 70.99,29.84 | 70.99,29.84 72.26,31.11 72.26,32.77 76.96,37.47 76.96,41.15 78.61,42.8 R7T.1 | 70.99,29.84 69.72,31.11 69.72,32.38 68.96,33.15 52.96,33.15 49.91,30.1 44.45,30.1 43.31,28.96 43.31,27.18 v45.09,25.4 | JSPI.3 22.35,26.8 25.02,24.13 26.92,24.13 SPI.5
  Top 0.61: R7.2 R7T.1
  Bottom 0.305: SPI.5 29.34,25.53 30.61,26.8 43.69,26.8 v45.09,25.4
MOSI  (via drill 0.41)
  Top 0.305: JTMOSI.2 70.99,27.3 | 70.99,27.3 72.26,28.57 72.26,29.84 72.9,30.48 74.17,30.48 74.8,31.11 74.8,34.29 78.49,37.97 R6T.1 | 70.99,27.3 69.72,28.57 69.72,29.84 69.09,30.48 52.83,30.48 51.69,29.34 44.58,29.34 44.07,28.83 44.07,27.94 v45.09,26.92
  Top 0.61: R6.2 R6T.1
  Bottom 0.305: JSPI.1 21.97,28.07 SPI.4 27.18,26.8 29.34,26.8 29.97,27.43 44.58,27.43 v45.09,26.92
N$2
  Bottom 0.305: JBUZ.2 10.62,42.55 BUZ.+
N$4
  Top 0.61: R1.2 R1T.2 79.38,13.21 Q1T.G 79.38,8.53 Q1.1
  Bottom 0.406: R1T.2 78.36,13.34 74.55,17.14 72.9,17.14 JTLED.2
N$5
  Top 0.203: SJ_DC.1 SJ_DC.2
  Top 0.305: JTDC.2 71.63,21.59 72.9,22.86 76.39,22.86 SJ_DC.2
  Top 0.61: R3.2 R3T.1 SJ_DC.1
N$10
  Top 0.813: 63.63,16.51 62.74,17.4 59.05,17.4 U1.2 | 63.63,16.51 63.63,12.45 | 63.63,12.45 63.63,9.22 U1.4 | U1T.VOUT 63.37,12.19 63.63,12.45 | 63.63,16.51 67.44,16.51 67.56,16.38 C1.+ C1T.+ 71.63,10.16 JPWR.1
OL
  Top 0.254: JP11.5 65.28,36.96 65.28,38.86
  Top 0.305: 65.28,38.86 68.83,42.42 68.83,48.26 76.33,55.75 77.72,55.75 JP24.5
OR
  Top 0.305: JP24.6 68.07,48.64 68.07,42.55 64.01,38.48 JP11.6
R+
  Top 0.406: JP11.4 69.85,41.53 69.85,47.88 73.28,51.31 78.87,51.31 81.79,54.23 JP24.4
R-
  Top 0.406: JP11.2 70.74,39.88 70.74,47.5 73.66,50.42 79.25,50.42 84.33,55.5 JP24.3
REF  (via drill 0.41)
  Top 0.305: JP8.14 28.45,43.05 29.59,41.91 40.39,41.91 42.8,39.5 53.34,39.5 v53.72,39.12
  Top 0.406: JP4.3 68.07,2.41 JP19.3
  Bottom 0.305: JP6.13 23.37,43.31 JP8.14 | JP4.3 68.07,6.73 63.63,11.18 63.63,25.78 62.61,26.8 58.04,26.8 54.74,30.1 54.74,32.89 53.72,33.91 v53.72,39.12
RST  (via drill 0.41)
  Top 0.305: RESET.3 3.17,19.99 3.17,25.78 9.53,32.13 22.35,32.13 25.15,29.34 26.92,29.34 28.19,30.61 SPI.1 | v35.81,30.23 35.81,25.78 JP7.5 | JP1.6 58.93,45.85 57.66,44.58 57.66,42.67 55.24,40.26 v49.15,40.26
  Top 0.813: RESET.4 RESET.3 | JP1.6 JP21.7
  Bottom 0.305: JP7.5 JP5.13 | SPI.1 28.83,30.23 v35.81,30.23 40.51,30.23 41.15,30.86 JP6.3 41.15,36.96 44.45,40.26 v49.15,40.26
SCK  (via drill 0.41)
  Top 0.305: R4T.1 78.87,27.94 72.9,27.94 72.26,27.3 72.26,26.16 71.5,25.4 70.99,25.4 | 70.99,25.4 70.36,25.4 69.72,26.04 69.72,27.3 69.09,27.94 67.82,27.94 66.04,29.72 53.09,29.72 51.94,28.57 v45.09,28.57 | JTSCK.2 70.99,25.4
  Top 0.61: R4.2 R4T.1
  Bottom 0.305: JSPI.5 27.05,29.34 SPI.3 44.58,28.07 v45.09,28.57
SCL
  Top 0.406: JP4.1 73.15,2.41 JP19.1
SDA
  Top 0.406: JP4.2 70.61,2.41 JP19.2
TFT_CS
  Top 0.406: TFT.12 87.63,17.91 D1T.A 84.33,17.14 R2T.2
  Top 0.61: R2.1 R2T.2 | D1.A D1T.A
TFT_DC
  Top 0.406: TFT.10 84.84,22.99 | 84.84,22.99 R3T.2 | 84.84,22.99 84.84,21.72 D2T.A
  Top 0.61: R3.1 R3T.2 | D2.A D2T.A
TFT_LED
  Top 0.61: Q1T.D 81.49,9.36 Q1.3
  Bottom 0.406: TFT.7 87.12,28.32 87.12,15.62 86.11,14.61 83.31,14.61 81.92,13.21 Q1T.D
TFT_MISO
  Top 0.406: R7T.2 84.33,41.78 D6T.A 87.5,40.39 | TFT.2 88.65,43.31 87.5,42.16 87.5,40.39 | TFT.6 87.5,35.05 87.5,40.39
  Top 0.61: R7.1 R7T.2 | D6.A D6T.A
TFT_MOSI
  Top 0.406: R6T.2 84.33,36.83 D5T.A 85.6,34.16 87.88,31.88 90.42,31.88 90.93,31.37 90.93,26.8 89.66,25.53 TFT.9
  Top 0.61: R6.1 R6T.2 | D5.A D5T.A
  Bottom 0.406: TFT.3 88.52,40.77 85.72,37.97 R6T.2
TFT_SCK
  Top 0.406: 84.58,28.07 84.58,26.92 D3T.A | TFT.8 84.58,28.07 | 84.58,28.07 R4T.2
  Top 0.61: R4.1 R4T.2 | D3.A D3T.A
  Bottom 0.406: TFT.5 90.81,35.69 91.44,35.05 91.44,28.7 90.81,28.07 TFT.8
TFT_T_CS
  Top 0.406: R5T.2 84.33,32 D4T.A
  Top 0.61: R5.1 R5T.2 | D4.A D4T.A
  Bottom 0.406: R5T.2 85.98,33.15 87.5,34.67 87.5,37.08 88.65,38.23 TFT.4
TFT_T_IRQ
  Top 0.406: TFT.1 86.23,45.85 D7T.A
  Top 0.61: D7T.A D7.A 82.49,46.8 R8T.2 R8.1
TFT_VCC
  Top 0.61: TFT.14 89.41,7.75 86.11,4.45 81.39,4.45 Q1.2 79.23,6.6 78.49,6.6 76.83,8.26 Q1T.S 76.83,11.94 76.07,12.7 JPWR.2
  Bottom 0.305: TFT.14 88.01,14.22 88.01,19.05 TFT.11
VIN  (via drill 0.81)
  Top 0.305: VINY.1 VINY.2 | VINX.1 VINX.2 31.62,23.62 JP7.2
  Top 0.61: VINX.1 31.62,28.57 v30.99,29.21 | v46.23,50.04 45.85,50.42 28.57,50.42 25.78,47.62 25.78,41.02 26.8,40.01 38.86,40.01 41.4,37.47 50.04,37.47 50.67,36.83 50.67,33.91 49.4,32.64 v48.51,32.64 48.46,32.7 VINY.2 | VINY.1 JP6.1
  Top 0.813: JP1.1 JP21.2
  Bottom 0.61: v30.99,29.21 43.31,29.21 45.85,31.75 47.62,31.75 v48.51,32.64 | v46.23,50.04 JP1.1
WAKE  (via drill 0.41)
  Top 0.254: SJ_T_IRQ.2 SJ_T_IRQ.1
  Top 0.305: JTMODE.2 70.99,32.51 76.33,37.85 76.33,42.04 v74.42,43.94 | v21.84,50.04 v11.43,50.04
  Top 0.406: SJ_T_IRQ.1 75.37,47.5 R8T.1 | v74.42,43.94 74.55,44.07 SJ_T_IRQ.2
  Top 0.61: R8.2 R8T.1
  Bottom 0.254: WAKE.3 1.68,31.9
  Bottom 0.305: v21.84,50.04 24.64,52.83 24.64,53.98 25.65,54.99 68.96,54.99 74.42,49.53 v74.42,43.94 | WAKE.3 1.68,46.38 4.19,48.9 10.29,48.9 v11.43,50.04
  Bottom 0.813: WAKE.3 WAKE.4

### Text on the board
tNames: PIRANHA | FISHINO | TFT SHIELD | OTHERS | OTHERS | PIRANHA | INT | DESIGNED BY MASSIMO DEL FEDELE | WWW.FISHINO.COM | EXT
bNames: A7 | A6 | A5 | A4 | A3 | A2 | A1 | A0 | D14 | VIN | GND | 5V | +3V3 | RES | IOREF | M2 | M1 | GND | IR | IL | OR | OL | R+ | R- | L+ | L- | PIRANHA | NANO / GUPPY | D0 | D1 | D2 | D3 | D4 | D5 | D6 | D7 | D8 | D9 | D10 | D11 | D12 | D13 | GND | REF | SDA | SCL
